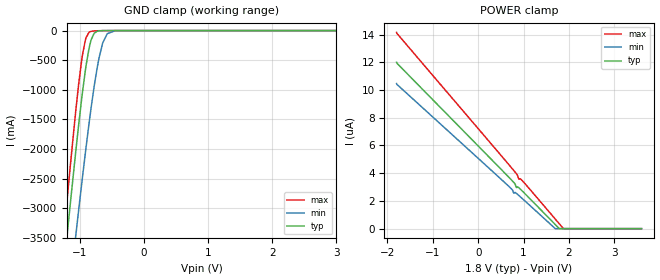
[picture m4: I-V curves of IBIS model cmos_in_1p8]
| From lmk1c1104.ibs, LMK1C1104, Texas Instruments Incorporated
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[Model]   cmos_in_1p8
Model_type   Input
Vinl = 0.54
Vinh = 1.26
|   typ   min   max
C_comp   7.121pF   6.747pF   7.634pF
[Voltage Range]   1.8   1.71   1.89
[Temperature Range]   25   150   -40
[Power Clamp Reference]   1.8   1.71   1.89
[GND Clamp Reference]   0   0   0
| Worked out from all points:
|   GND clamp passes 1 mA (typ) near -0.65 V on its own axis
[GND Clamp]
|   Voltage   I(typ)   I(min)   I(max)
-1.8V     -10.22A    -10.92A    -10.14A
-1.438V   -6.13A     -7.231A    -5.731A
-1.211V   -3.633A    -4.944A    -3.043A
-1.184V   -3.342A    -4.676A    -2.732A
-1.06V    -2.042A    -3.462A    -1.358A
-957.6mV  -1.059A    -2.494A    -424mA
-903.6mV  -621.2mA   -2.006A    -134.4mA
-838.8mV  -233.2mA   -1.45A     -20.86mA
-725.4mV  -10.63mA   -625.2mA   -3.216mA
-644.4mV  -919.7uA   -225.7mA   -839.1uA
-444.6mV  -5.476uA   -2.254mA   -5.113uA
3.6V      0A         0A         0A
[POWER Clamp]
|   Voltage   I(typ)   I(min)   I(max)
-1.8V     11.99uA    10.46uA    14.15uA
689.4mV   3.659uA    3.007uA    4.563uA
754.2mV   3.439uA    2.794uA    4.312uA
781.2mV   3.344uA    2.579uA    4.206uA
813.6mV   3.211uA    2.608uA    4.079uA
840.6mV   2.979uA    2.547uA    3.968uA
894.6mV   2.957uA    2.395uA    3.599uA
981mV     2.684uA    2.142uA    3.43uA
1.694V    312.4nA    9.789nA    710.6nA
1.786V    5.915nA    0A         358.1nA
1.877V    0A         0A         5.414nA
3.6V      0A         0A         0A
